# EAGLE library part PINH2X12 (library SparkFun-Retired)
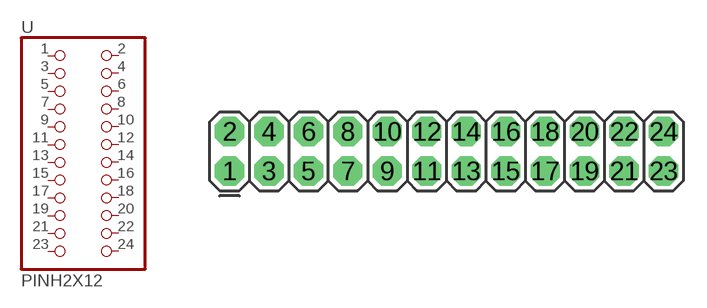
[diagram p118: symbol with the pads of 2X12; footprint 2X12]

Designator prefix -

## PINH2X12  [2X12]
1  1  pas
2  2  pas
3  3  pas
4  4  pas
5  5  pas
6  6  pas
7  7  pas
8  8  pas
9  9  pas
10  10  pas
11  11  pas
12  12  pas
13  13  pas
14  14  pas
15  15  pas
16  16  pas
17  17  pas
18  18  pas
19  19  pas
20  20  pas
21  21  pas
22  22  pas
23  23  pas
24  24  pas

## Footprint 2X12 (pad centres in mm)
drill 1.016 pad 1.88 octagon: 1 0,0; 2 0,2.54; 3 2.54,0; 4 2.54,2.54; 5 5.08,0; 6 5.08,2.54; 7 7.62,0; 8 7.62,2.54; 9 10.16,0; 10 10.16,2.54; 11 12.7,0; 12 12.7,2.54; 13 15.24,0; 14 15.24,2.54; 15 17.78,0; 16 17.78,2.54; 17 20.32,0; 18 20.32,2.54; 19 22.86,0; 20 22.86,2.54; 21 25.4,0; 22 25.4,2.54; 23 27.94,0; 24 27.94,2.54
